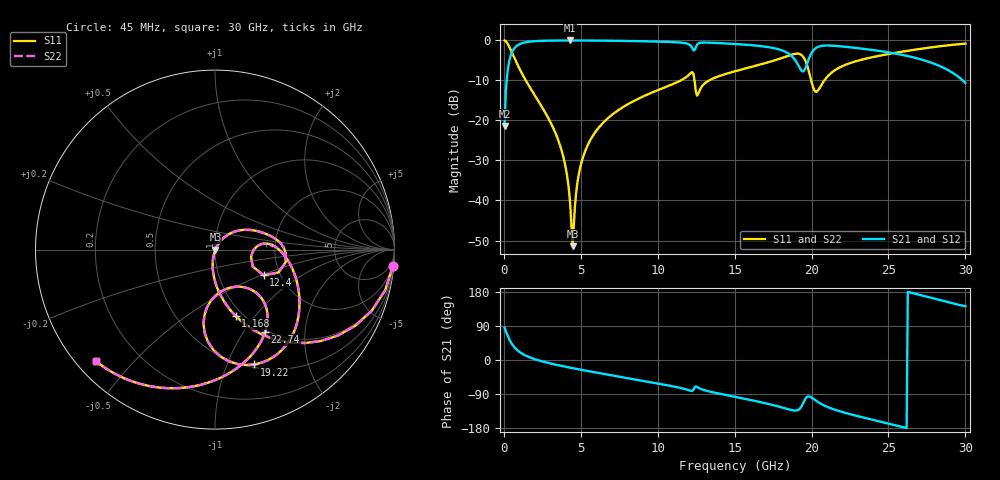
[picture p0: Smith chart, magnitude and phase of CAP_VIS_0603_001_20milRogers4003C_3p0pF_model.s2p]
! S-parameter model data by Modelithics Inc.  support@modelithics.com  813-866-6335  Tampa FL USA
! S-Parameter data specifications:
! Substrate: 20-mil Rogers 4003C, substrate thickness, H=0.508mm, Dielectric constant, Er=3.75
! PCB Mounting Pad Footprint: Pad width, PadW=0.90mm , Pad length, PadL=1.00mm , Pad gap, PadG (edge-to-edge)=1.00mm , Reference planes=3.0mm apart
! Created Wed Nov 18 13:21:31 2015
# hz S ma R 50
! 2 Port Network Data from SP1.SP block
! freq  magS11  angS11  magS21  angS21  magS12  angS12  magS22  angS22
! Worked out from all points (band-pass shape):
!   401 points, 45 MHz to 30 GHz, reference 50 ohm
!   highest |S21| = -0.03 dB at 4.314 GHz (marker M1); lowest = -21.4 dB at 45 MHz (marker M2)
!   |S21| within 3 dB of the highest: 520.3 MHz to 18.38 GHz (17.86 GHz wide, 189 % of centre); 20.02 GHz to 25.04 GHz (5.018 GHz wide, 22.3 % of centre)
!   lowest |S11| = -51.4 dB at 4.463 GHz (marker M3), VSWR 1.01, Z = 50.2 - j0.111 ohm
!   |S11| at or under -10 dB: 1.421 GHz to 11.5 GHz (10.08 GHz wide, 156 % of centre); 12.39 GHz to 13.34 GHz (947.8 MHz wide, 7.37 % of centre); 19.97 GHz to 20.83 GHz (860.9 MHz wide, 4.22 % of centre)
!   |S22| runs from -51.4 to 0.0 dB; largest |S21 - S12| = 0
!   S11 on the Smith chart (normalised r, x): 45 MHz: 1, -22; 1.168 GHz: 0.92, -0.80; 12.4 GHz: 1.64, -0.52; 19.22 GHz: 0.53, -1.25; 22.74 GHz: 0.97, -1.26; 30 GHz: 0.05, -0.39
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4.5e7  0.9964 -5.1  0.08522 84.9  0.08522 84.9  0.9964 -5.1
4.194375e8  0.7791 -40.8  0.6264 49.2  0.6264 49.2  0.7791 -40.8
1.168312e9  0.3871 -72.7  0.9206 17.1  0.9206 17.1  0.3871 -72.7
3.564712e9  0.05446 -101.6  0.9958 -14.1  0.9958 -14.1  0.05446 -101.6
4.014038e9  0.02586 -102.2  0.9968 -17.9  0.9968 -17.9  0.02586 -102.2
4.313588e9  0.00879 -92.9  0.997 -20.3  0.997 -20.3  0.00879 -92.9
4.463362e9  0.002688 -24.3  0.9969 -21.5  0.9969 -21.5  0.002688 -24.3
5.062462e9  0.03082 58.5  0.9962 -26.2  0.9962 -26.2  0.03082 58.5
6.6351e9  0.1013 50.3  0.9909 -37.8  0.9909 -37.8  0.1013 50.3
1.007992e10  0.2419 26.2  0.9643 -62.6  0.9643 -62.6  0.2419 26.2
1.217678e10  0.3954 -3.2  0.8412 -81.6  0.8412 -81.6  0.3954 -3.2
1.240144e10  0.3066 -27.9  0.7567 -72.3  0.7567 -72.3  0.3066 -27.9
1.26261e10  0.214 -0.9  0.9112 -72.7  0.9112 -72.7  0.214 -0.9
1.50225e10  0.4109 -8.5  0.9006 -97.1  0.9006 -97.1  0.4109 -8.5
1.809289e10  0.6036 -40.1  0.7473 -125.4  0.7473 -125.4  0.6036 -40.1
1.92162e10  0.676 -71.2  0.4592 -129.3  0.4592 -129.3  0.676 -71.2
2.003996e10  0.2828 -94.2  0.7163 -100.2  0.7163 -100.2  0.2828 -94.2
2.108839e10  0.3623 -46.1  0.862 -124.9  0.862 -124.9  0.3623 -46.1
2.273591e10  0.5376 -58.7  0.8102 -145.4  0.8102 -145.4  0.5376 -58.7
2.505742e10  0.6782 -80.7  0.7048 -168.4  0.7048 -168.4  0.6782 -80.7
2.782826e10  0.8195 -109.7  0.5222 163.6  0.5222 163.6  0.8195 -109.7
3e10  0.9092 -136.9  0.2934 141.8  0.2934 141.8  0.9092 -136.9
